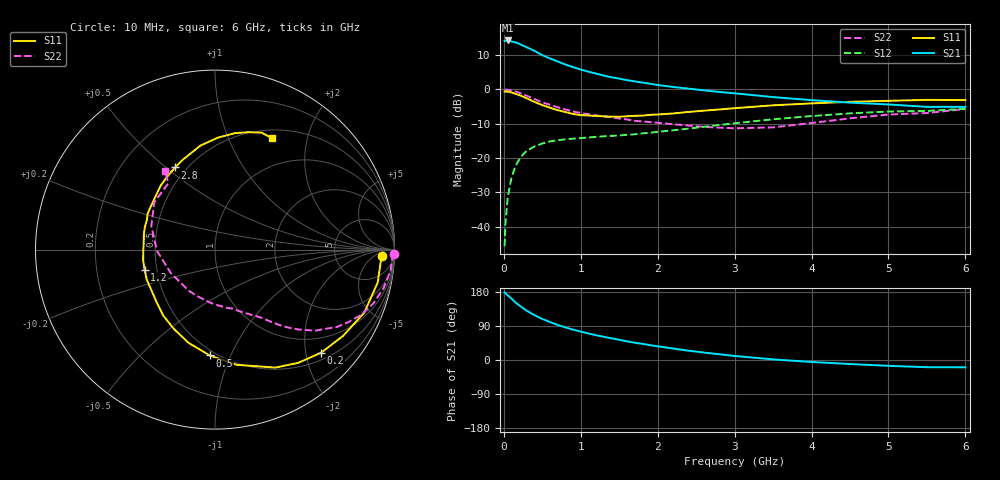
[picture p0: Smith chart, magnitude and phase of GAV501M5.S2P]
! Infineon Technologies  Discrete & RF Semiconductors
! BF775
! Si NPN RF Bipolar Junction Transistor in SOT23
! VCE = 0.5 V  IC = 1.5 mA
! Common Emitter S-Parameters:  May  1996
# GHz  S  MA  R  50
!  f  S11  S21  S12  S22
! GHz  MAG  ANG  MAG  ANG  MAG  ANG  MAG  ANG
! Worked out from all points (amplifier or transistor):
!   36 points, 10 MHz to 6 GHz, reference 50 ohm
!   highest |S21| = 14.2 dB at 50 MHz (marker M1)
!   |S21| within 3 dB of that: start of sweep to 396.1 MHz
!   unconditionally stable (mu >= 1): 1.12 GHz to end of sweep
!   at 250 MHz: K = 0.27, MSG = 15.8 dB, |S12| = -19.0 dB
!   at 1.4 GHz: K = 1.16, MAG = 6.1 dB, |S12| = -13.6 dB
!   at 6 GHz: K = 1.11, MAG = -1.8 dB, |S12| = -5.7 dB
!   S11 on the Smith chart (normalised r, x): 10 MHz: 21, -12; 200 MHz: 0.64, -2.31; 500 MHz: 0.46, -0.84; 1.2 GHz: 0.43, -0.11; 2.8 GHz: 0.44, +0.54; 6 GHz: 0.60, +1.45
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0.01  0.9308 -2.3  5.05 178.6  0.0052 89.3  0.9951 -1.3
0.02  0.9254 -4.6  5.068 176.2  0.0107 85.3  0.9886 -2.5
0.05  0.9249 -11.4  5.147 170.7  0.0267 82.5  0.9859 -6.6
0.1  0.9029 -22.9  4.975 161.9  0.052 76.0  0.9635 -12.9
0.15  0.8603 -34.0  4.838 152.1  0.0755 69.2  0.9319 -18.8
0.2  0.8241 -44.2  4.621 144.2  0.0952 63.4  0.8911 -24.1
0.3  0.7385 -62.9  4.085 129.8  0.1274 54.0  0.8052 -32.3
0.4  0.653 -79.4  3.627 118.3  0.1478 46.6  0.7177 -39.0
0.5  0.5903 -92.9  3.148 108.3  0.1626 41.2  0.6461 -43.6
0.6  0.5398 -105.9  2.81 100.1  0.1741 37.0  0.5948 -46.9
0.7  0.4974 -117.5  2.543 92.6  0.1816 34.3  0.549 -49.7
0.8  0.4671 -128.2  2.298 86.0  0.1869 32.0  0.5095 -52.2
0.9  0.4373 -138.2  2.104 80.1  0.1913 30.8  0.4763 -54.4
1.1  0.4155 -156.3  1.809 70.0  0.1991 28.7  0.4335 -58.6
1.2  0.4081 -164.1  1.694 65.3  0.203 27.9  0.4178 -60.8
1.6  0.4052 168.2  1.359 49.3  0.2176 28.3  0.3641 -69.4
2.2  0.4448 138.2  1.082 30.3  0.253 29.9  0.3106 -87.2
2.8  0.5086 115.9  0.916 15.2  0.3021 28.8  0.2767 -113.1
3.5  0.5851 98.0  0.771 1.6  0.3661 23.6  0.279 -152.3
4.5  0.6577 80.4  0.64 -10.6  0.4464 12.4  0.3783 159.7
5.5  0.7016 68.2  0.555 -19.0  0.4842 -0.8  0.4518 125.1
6  0.6969 63.1  0.555 -19.2  0.5199 -4.4  0.5174 122.5
